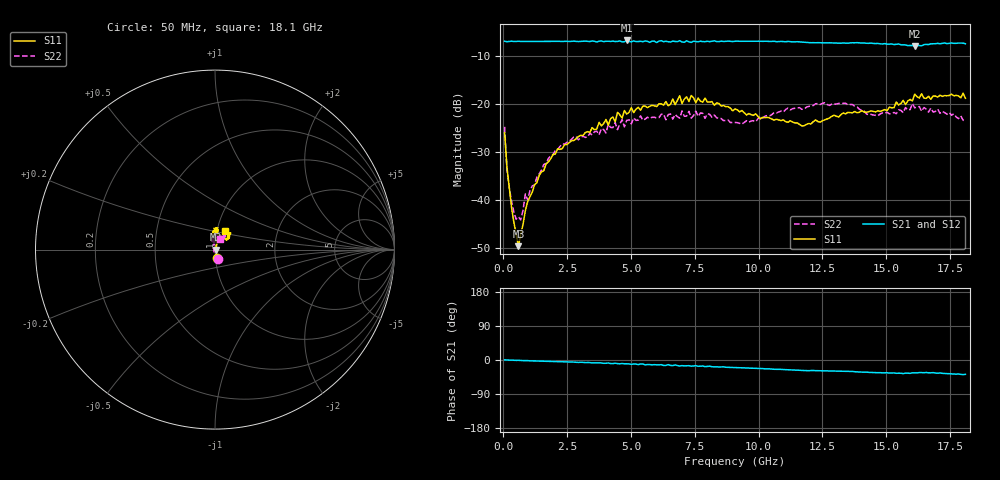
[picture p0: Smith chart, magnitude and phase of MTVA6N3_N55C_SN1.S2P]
! Network Analyzer HP8720D.06.14 Serial No. US36140669
!  5 Jul 2005  09:49:00
! Frequency  S11  S21  S12  S22
# HZ  S  DB R 50
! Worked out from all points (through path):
!   201 points, 50 MHz to 18.1 GHz, reference 50 ohm
!   highest |S21| = -6.81 dB at 4.833 GHz (marker M1); lowest = -8.0 dB at 16.11 GHz (marker M2)
!   group delay of S21, straight-line fit = 6.09 ps
!   lowest |S11| = -49.5 dB at 591.5 MHz (marker M3), VSWR 1.01, Z = 50.3 + j0.0132 ohm
!   |S11| at or under -10 dB: start of sweep to end of sweep
!   |S22| runs from -44.1 to -19.7 dB; largest |S21 - S12| = 0.015
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5e7  -25.98 -75.9  -6.98 0.4  -6.99 0.5  -24.74 -71.2
1.4025e8  -33.02 -68.6  -7.07 0.0  -7.05 0.0  -33.56 -95.9
2.305e8  -37.16 -61.4  -7.01 -0.2  -7.01 -0.2  -37.33 -112.1
5.0125e8  -47.02 -23.1  -7.02 -1.0  -7.02 -0.9  -43.91 -163.3
5.915e8  -49.52 2.2  -6.98 -0.9  -7.04 -0.9  -43.41 180.0
6.8175e8  -47.09 27.3  -7.01 -1.3  -7.03 -1.3  -44.05 160.7
8.6225e8  -42.16 47.2  -7.00 -1.5  -7.04 -1.5  -38.69 146.8
9.525e8  -40.26 53.3  -7.01 -1.7  -7.01 -1.8  -39.93 129.9
1.40375e9  -34.86 64.7  -7.00 -2.8  -7.02 -2.8  -34.51 110.3
2.30625e9  -29.27 73.1  -7.03 -4.6  -7.02 -4.6  -28.27 99.8
3.1185e9  -26.53 81.3  -7.00 -6.2  -7.03 -6.4  -26.67 108.9
4.83325e9  -22.11 85.6  -6.81 -9.9  -6.94 -10.7  -23.41 95.2
6.09675e9  -19.97 83.4  -6.95 -13.0  -6.89 -13.0  -22.83 94.9
6.909e9  -18.29 87.8  -6.85 -15.8  -6.98 -15.0  -22.94 86.1
6.99925e9  -19.92 87.2  -7.13 -14.8  -7.17 -16.0  -21.46 88.2
7.36025e9  -18.23 82.2  -7.22 -16.2  -7.07 -15.5  -22.93 92.1
7.54075e9  -19.74 82.7  -7.04 -15.1  -6.94 -16.8  -21.51 91.8
9.075e9  -21.04 96.3  -6.97 -19.8  -6.96 -19.9  -23.84 73.3
1.21435e10  -23.65 70.5  -7.27 -27.6  -7.23 -28.0  -20.31 61.3
1.512175e10  -20.66 40.3  -7.59 -34.5  -7.47 -34.4  -22.05 61.2
1.61145e10  -17.96 46.3  -8.00 -33.8  -7.77 -34.3  -20.79 56.7
1.81e10  -18.81 61.7  -7.50 -37.8  -7.56 -38.8  -23.57 67.4
